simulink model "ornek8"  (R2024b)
settings: Solver=VariableStepAuto  StartTime=0.0  StopTime=0.04  RelTol=1e-3

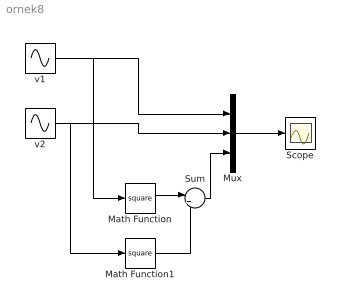
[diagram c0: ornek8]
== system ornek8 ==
  Math Function : Math  Operator=square
  Math Function1 : Math  Operator=square
  Mux : Mux  Inputs=3
  Scope : Scope
  Sum : Sum  Inputs=|++
  v1 : Sin  Frequency=100*pi  SampleTime=0
  v2 : Sin  Frequency=100*pi  Phase=pi/2  SampleTime=0
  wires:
  Mux/1 -> Scope/1
  v1/1 -> Math Function/1, Mux/1
  v2/1 -> Math Function1/1, Mux/2
  Math Function/1 -> Sum/1
  Math Function1/1 -> Sum/2
  Sum/1 -> Mux/3
